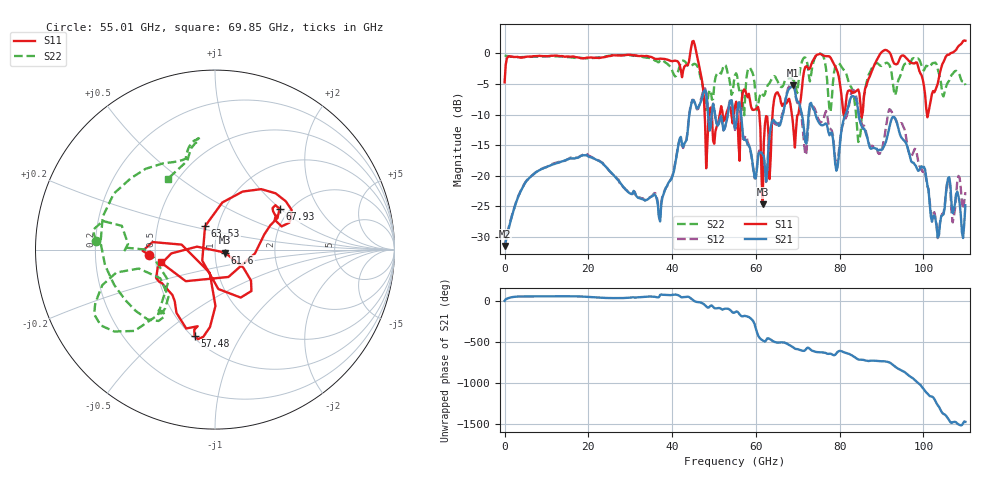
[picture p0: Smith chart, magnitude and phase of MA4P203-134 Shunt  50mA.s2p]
!Keysight Technologies,N5247B,US61255204,A.15.70.20
!Date: Friday, October 21, 2022 15:24:17
!Correction: S11(C  4-Port  )
!S31(C  4-Port  )
!S13(C  4-Port  )
!S33(C  4-Port  )
!S2P File: Measurements: S11, S31, S13, S33:
# Hz S  dB  R 50
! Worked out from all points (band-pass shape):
!   401 points, 10 MHz to 110 GHz, reference 50 ohm
!   highest |S21| = -5.19 dB at 68.75 GHz (marker M1); lowest = -31.5 dB at 10 MHz (marker M2)
!   |S21| within 3 dB of the highest: 66.94 GHz to 70.34 GHz (3.405 GHz wide, 4.96 % of centre); 82.2 GHz to 84.15 GHz (1.945 GHz wide, 2.34 % of centre)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
!   lowest |S11| = -24.7 dB at 61.6 GHz (marker M3), VSWR 1.12, Z = 55.9 - j1.86 ohm
!   |S11| at or under -10 dB: 49.45 GHz to 51.36 GHz (1.911 GHz wide, 3.79 % of centre); 60.83 GHz to 63.96 GHz (3.137 GHz wide, 5.03 % of centre); 68.59 GHz to 70.1 GHz (1.515 GHz wide, 2.18 % of centre)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
!   |S22| runs from -14.5 to 0.0 dB; largest |S21 - S12| = 0.17
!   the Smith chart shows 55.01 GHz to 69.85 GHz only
!   S11 on the Smith chart (normalised r, x): 55.01 GHz: 0.46, -0.03; 57.48 GHz: 0.51, -0.65; 61.6 GHz: 1.12, -0.04; 63.53 GHz: 0.87, +0.23; 67.93 GHz: 1.77, +0.99; 69.85 GHz: 0.53, -0.08
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1e7  -4.72 -180.0  -31.47 -4.3  -31.52 -4.3  -0.39 179.9
1.843332e10  -0.80 145.7  -16.70 48.1  -16.68 47.9  -0.74 145.3
3.685665e10  -0.89 154.7  -26.79 40.9  -26.44 41.5  -1.43 154.3
4.51059e10  2.04 85.2  -7.64 0.0  -7.60 -2.2  -1.74 115.4
4.813062e10  -18.77 59.3  -6.57 -71.2  -6.39 -71.6  -9.23 113.1
5.5005e10  -8.62 -175.7  -12.27 -142.6  -12.52 -144.2  -3.53 175.7
5.747978e10  -6.11 -103.2  -14.10 172.9  -13.47 178.3  -6.31 -131.1
6.16044e10  -24.70 -16.5  -16.55 -122.6  -16.64 -120.6  -6.73 -132.8
6.352922e10  -16.99 113.1  -12.05 -113.3  -12.43 -110.2  -4.51 -160.8
6.792882e10  -7.42 32.3  -5.78 -178.7  -5.38 180.0  -4.10 99.1
6.875375e10  -10.84 17.1  -5.19 158.3  -4.92 154.4  -4.27 98.7
6.985365e10  -10.14 -167.0  -7.80 131.5  -8.08 131.0  -6.48 123.4
7.342832e10  -1.38 178.4  -8.66 112.3  -8.65 107.8  -2.26 156.3
7.645305e10  -0.43 -165.5  -11.52 87.4  -9.93 119.1  -1.28 148.2
7.947778e10  -3.00 -147.4  -18.64 96.3  -17.83 94.9  -1.64 -137.1
8.415235e10  -6.04 -39.1  -8.20 13.2  -7.75 18.2  -12.24 -169.7
8.745205e10  -3.24 49.8  -15.60 -8.3  -15.23 5.3  -2.71 53.7
9.185165e10  0.21 88.7  -12.09 -30.2  -9.12 -22.7  -1.90 76.3
9.79011e10  -1.64 173.3  -18.16 119.0  -15.60 116.9  -0.87 -177.0
1.023007e11  -6.15 -66.3  -26.67 -93.0  -26.21 -86.1  -1.55 -116.4
1.058754e11  -0.23 -7.5  -20.41 9.5  -20.73 5.0  -4.70 -38.3
1.1e11  2.08 46.2  -24.81 -29.2  -22.68 -27.2  -5.18 10.6
